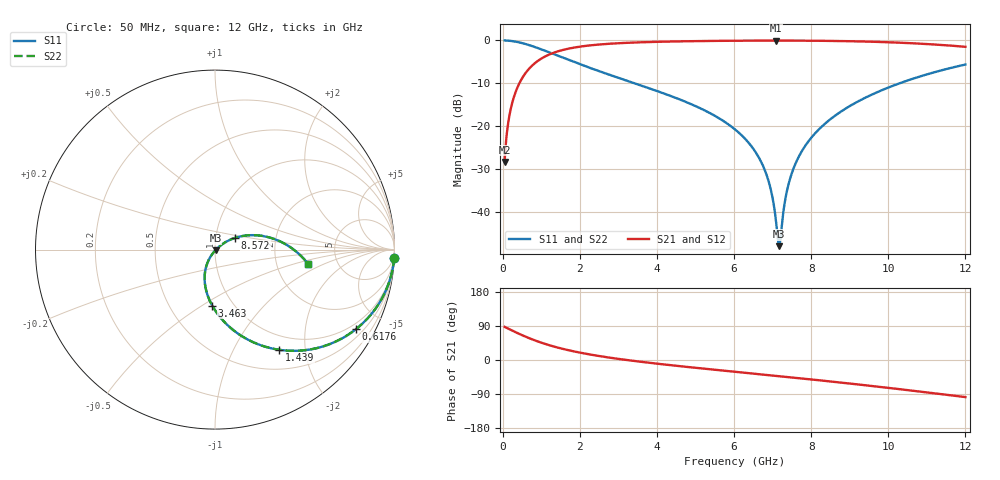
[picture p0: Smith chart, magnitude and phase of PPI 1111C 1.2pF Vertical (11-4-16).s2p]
# GHz S MA R 50
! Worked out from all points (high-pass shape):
!   1601 points, 50 MHz to 12 GHz, reference 50 ohm
!   highest |S21| = -0.04 dB at 7.078 GHz (marker M1); lowest = -28.3 dB at 50 MHz (marker M2)
!   |S21| within 3 dB of the highest: 1.272 GHz to end of sweep
!   lowest |S11| = -47.8 dB at 7.168 GHz (marker M3), VSWR 1.01, Z = 50.3 - j0.287 ohm
!   |S11| at or under -10 dB: 3.431 GHz to 10.28 GHz (6.852 GHz wide, 99.9 % of centre)
!   |S22| runs from -47.8 to 0.0 dB; largest |S21 - S12| = 0
!   S11 on the Smith chart (normalised r, x): 50 MHz: 1, -45; 617.6 MHz: 0.77, -3.65; 1.439 GHz: 0.77, -1.54; 3.463 GHz: 0.80, -0.55; 8.572 GHz: 1.24, +0.16; 12 GHz: 3.04, -0.67
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0.05  0.9992 -2.5  0.03864 87.5  0.03864 87.5  0.9992 -2.5
0.1545625  0.9929 -7.8  0.1187 82.2  0.1187 82.2  0.9929 -7.8
0.259125  0.9804 -13.0  0.1966 77.0  0.1966 77.0  0.9804 -13.0
0.617625  0.9017 -29.5  0.4318 60.5  0.4318 60.5  0.9017 -29.5
0.9835938  0.7934 -43.6  0.6077 46.3  0.6077 46.3  0.7934 -43.6
1.439188  0.662 -57.4  0.7482 32.5  0.7482 32.5  0.662 -57.4
2.044156  0.5212 -71.2  0.8518 18.7  0.8518 18.7  0.5212 -71.2
3.463219  0.3127 -92.8  0.9474 -3.2  0.9474 -3.2  0.3127 -92.8
4.038312  0.2548 -99.5  0.9642 -10.1  0.9642 -10.1  0.2548 -99.5
6.025  0.09237 -118.9  0.992 -31.1  0.992 -31.1  0.09237 -118.9
6.742  0.0356 -122.2  0.9952 -38.3  0.9952 -38.3  0.0356 -122.2
6.943656  0.01927 -118.6  0.9955 -40.3  0.9955 -40.3  0.01927 -118.6
7.078094  0.008664 -104.2  0.9956 -41.7  0.9956 -41.7  0.008664 -104.2
7.167719  0.004058 -44.7  0.9956 -42.6  0.9956 -42.6  0.004058 -44.7
7.212531  0.005474 -1.3  0.9955 -43.1  0.9955 -43.1  0.005474 -1.3
7.346969  0.0157 30.2  0.9953 -44.5  0.9953 -44.5  0.0157 30.2
7.481406  0.02713 35.1  0.995 -45.9  0.995 -45.9  0.02713 35.1
7.705469  0.04683 36.4  0.9941 -48.2  0.9941 -48.2  0.04683 36.4
8.019156  0.07542 35.0  0.9921 -51.5  0.9921 -51.5  0.07542 35.0
8.571844  0.1286 30.4  0.9863 -57.4  0.9863 -57.4  0.1286 30.4
10.01331  0.2846 15.1  0.9521 -73.7  0.9521 -73.7  0.2846 15.1
12  0.5247 -8.7  0.8432 -97.9  0.8432 -97.9  0.5247 -8.7
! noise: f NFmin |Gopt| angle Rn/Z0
0.05  0.0008574  0.9629  2.059  0.005225
1.372  0.004531  0.7281  11.35  0.003284
2.701  0.007314  0.6778  18.79  0.004271
4.031  0.009854  0.6545  26.21  0.005165
5.36  0.01234  0.6453  33.41  0.006071
6.682  0.01487  0.6459  40.23  0.007059
8.012  0.01756  0.6541  46.72  0.008213
9.341  0.0205  0.6683  52.85  0.00961
10.67  0.02379  0.6874  58.62  0.01136
12  0.02757  0.7104  64.09  0.01362
